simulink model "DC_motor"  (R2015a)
settings: Solver=ode15s  StartTime=0.0  StopTime=10.0  RelTol=1e-3
libraries: fl_lib x13, nesl_utility x3

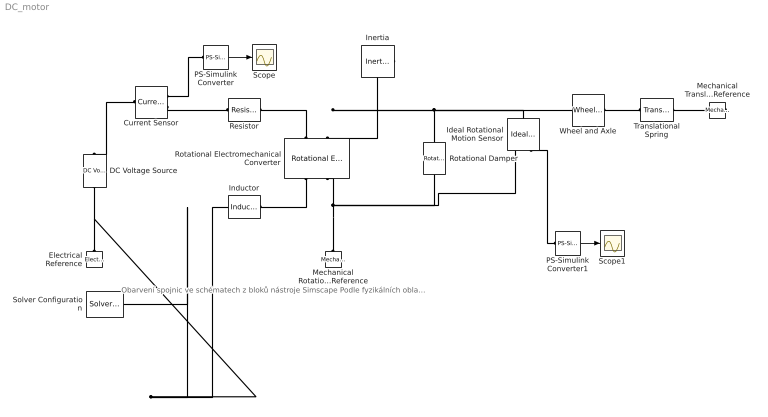
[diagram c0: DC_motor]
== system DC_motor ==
  note: Obarvení spojnic ve schématech z bloků nástroje Simscape Podle fyzikálních oblastí. V tomto modelu najdeme oblast elektrickou (modrá), mechanickou rotační (žlutozelená), mechanickou translační (zelená) a fyzikální signály (hnědá).
  Current Sensor : fl_lib/Electrical/Electrical Sensors/Current Sensor
  DC Voltage Source : fl_lib/Electrical/Electrical Sources/DC Voltage Source  v0=1 V
  Electrical Reference : fl_lib/Electrical/Electrical Elements/Electrical Reference
  Ideal Rotational Motion Sensor : fl_lib/Mechanical/Mechanical Sensors/Ideal Rotational Motion Sensor  offset=0 rad
  Inductor : fl_lib/Electrical/Electrical Elements/Inductor  l=1e-6 H  r=0 Ohm  g=1e-9 1/Ohm  i_specify=off  i_priority=High  i=0 A  v_specify=off  v_priority=High  v=0 V  i_L_specify=off  i_L_priority=High  i_L=0 A
  Inertia : fl_lib/Mechanical/Rotational Elements/Inertia  inertia=0.01 kg*m^2  w_specify=off  w_priority=High  w=0 rad/s  t_specify=off  t_priority=High  t=0 N*m
  Mechanical Rotational Reference : fl_lib/Mechanical/Rotational Elements/Mechanical Rotational Reference
  Mechanical Translational Reference : fl_lib/Mechanical/Translational Elements/Mechanical Translational Reference
  PS-Simulink Converter : nesl_utility/PS-Simulink Converter  PhysicalDomain=network_engine_domain  SubClassName=ps_output  LeftPortType=input  RightPortType=output  PseudoPeriodic=off  Frequencies=[]  Unit=A  AffineConversion=off
  PS-Simulink Converter1 : nesl_utility/PS-Simulink Converter  PhysicalDomain=network_engine_domain  SubClassName=ps_output  LeftPortType=input  RightPortType=output  PseudoPeriodic=off  Frequencies=[]  Unit=deg  AffineConversion=off
  Resistor : fl_lib/Electrical/Electrical Elements/Resistor  R=1 Ohm  i_specify=off  i_priority=High  i=0 A  v_specify=off  v_priority=High  v=0 V
  Rotational Damper : fl_lib/Mechanical/Rotational Elements/Rotational Damper  D=0.001 N*m/(rad/s)  w_specify=off  w_priority=High  w=0 rad/s  t_specify=off  t_priority=High  t=0 N*m
  Rotational Electromechanical Converter : fl_lib/Electrical/Electrical Elements/Rotational Electromechanical Converter  K=0.1 V/(rad/s)  i_specify=off  i_priority=High  i=0 A  v_specify=off  v_priority=High  v=0 V  t_specify=off  t_priority=High  t=0 N*m  w_specify=off  w_priority=High  w=0 rad/s
  Scope : Scope
  Scope1 : Scope
  Solver Configuration : nesl_utility/Solver Configuration  PhysicalDomain=network_engine_domain  SubClassName=solver  LeftPortType=input  RightPortType=generic  Accelerate=off  Tones=[]  Harmonics=[]  SimulateNoise=off  Profile=off  UseLocalSampling=off  EnableSwitchedLinearOptims=on  FrequencyDomain=off  UseCCode=off  RelTol=0.001  AbsTol=1e-06  MinStep=1e-09  ToWorkspace=off  RevertToSquareIcSolve=off  NumHomotopyIterations=100  DoDC=off  ResidualTolerance=1e-09  UseLocalSolver=off  LocalSolverChoice=NE_BACKWARD_EULER_ADVANCER  LocalSolverSampleTime=0.001  DoFixedCost=off  MaxNonlinIter=3  MaxModeIter=2  LinearAlgebra=Sparse  DelaysMemoryBudget=1024  AutomaticFiltering=on  FilteringTimeConstant=0.001
  Translational Spring : fl_lib/Mechanical/Translational Elements/Translational Spring  spr_rate=10 N/m  v_specify=off  v_priority=High  v=0 m/s  f_specify=off  f_priority=High  f=0 N  x_specify=off  x_priority=High  x=0 m
  Wheel and Axle : fl_lib/Mechanical/Mechanisms/Wheel and Axle  R=0.05 m  or=1  orient=1  t_specify=off  t_priority=High  t=0 N*m  f_specify=off  f_priority=High  f=0 N
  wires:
  PS-Simulink Converter/1 -> Scope/1
  PS-Simulink Converter1/1 -> Scope1/1
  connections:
  Electrical Reference/LConn1 -- Solver Configuration/RConn1 -- Inductor/LConn1 -- DC Voltage Source/RConn1
  Current Sensor/RConn2 -- Resistor/LConn1
  Current Sensor/LConn1 -- DC Voltage Source/LConn1
  PS-Simulink Converter/LConn1 -- Current Sensor/RConn1
  Rotational Electromechanical Converter/LConn1 -- Resistor/RConn1
  Rotational Electromechanical Converter/RConn1 -- Inductor/RConn1
  Inertia/LConn1 -- Ideal Rotational Motion Sensor/LConn1 -- Wheel and Axle/LConn1 -- Rotational Damper/LConn1 -- Rotational Electromechanical Converter/LConn2
  Mechanical Rotational Reference/LConn1 -- Ideal Rotational Motion Sensor/RConn1 -- Rotational Damper/RConn1 -- Rotational Electromechanical Converter/RConn2
  PS-Simulink Converter1/LConn1 -- Ideal Rotational Motion Sensor/RConn3
  Translational Spring/LConn1 -- Wheel and Axle/RConn1
  Mechanical Translational Reference/LConn1 -- Translational Spring/RConn1
